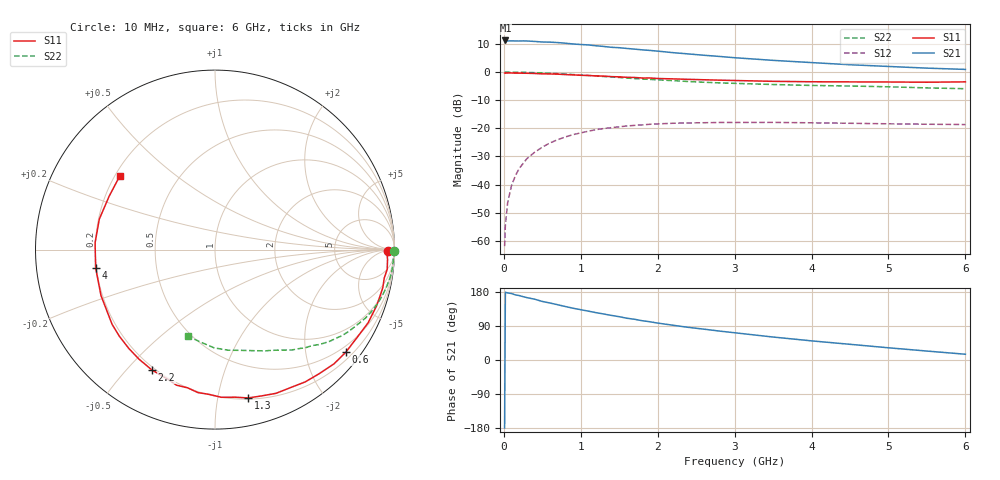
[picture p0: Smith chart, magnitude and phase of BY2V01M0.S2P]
! SIEMENS Small Signal Semiconductors
! BFY420
! Si NPN RF SIEGET Grounded Emitter Transistor in MICRO-X
! VCE = 2 V  IC = 1 mA
! Common Emitter S-Parameters:  October  1996
# GHz  S  MA  R  50
!  f  S11  S21  S12  S22
! GHz  MAG  ANG  MAG  ANG  MAG  ANG  MAG  ANG
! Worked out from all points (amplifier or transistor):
!   36 points, 10 MHz to 6 GHz, reference 50 ohm
!   highest |S21| = 11.3 dB at 20 MHz (marker M1)
!   |S21| within 3 dB of that: start of sweep to 1.666 GHz
!   unconditionally stable (mu >= 1): 4.55 GHz to end of sweep
!   at 250 MHz: K = 0.05, MSG = 21.8 dB, |S12| = -32.5 dB
!   at 1.4 GHz: K = 0.21, MSG = 14.3 dB, |S12| = -19.8 dB
!   at 6 GHz: K = 1.33, MAG = 6.4 dB, |S12| = -18.7 dB
!   S11 on the Smith chart (normalised r, x): 10 MHz: 48, -13; 600 MHz: 0.36, -2.86; 1.3 GHz: 0.21, -1.23; 2.2 GHz: 0.19, -0.59; 4 GHz: 0.20, -0.07; 6 GHz: 0.22, +0.32
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0.01  0.9622 -0.6  3.652 -179.3  0.0008 102.8  0.9999 -0.4
0.02  0.9583 -1.4  3.654 178.7  0.0019 88.0  0.9964 -0.6
0.05  0.9628 -3.2  3.583 177.0  0.0048 86.9  0.9983 -1.6
0.1  0.9657 -6.5  3.595 175.4  0.0096 85.8  0.9941 -3.2
0.15  0.9561 -9.6  3.579 171.8  0.0143 83.1  0.9947 -4.9
0.2  0.9588 -12.8  3.574 170.0  0.0193 81.8  0.9936 -6.3
0.3  0.9531 -19.2  3.574 164.6  0.0289 78.7  0.9866 -9.5
0.4  0.9457 -25.5  3.511 160.5  0.0374 74.2  0.977 -12.6
0.5  0.9306 -31.9  3.432 154.5  0.0462 70.5  0.9663 -15.6
0.6  0.9262 -38.1  3.409 150.4  0.055 67.0  0.9535 -18.6
0.8  0.9027 -50.0  3.265 141.1  0.0702 59.3  0.9222 -24.3
1.1  0.8699 -67.0  3.041 128.9  0.0889 49.8  0.8708 -31.8
1.3  0.8469 -77.4  2.858 121.3  0.0991 43.8  0.8347 -36.3
1.6  0.807 -92.4  2.633 110.2  0.1101 35.9  0.7835 -42.5
1.8  0.7851 -101.2  2.484 103.6  0.1151 31.2  0.7531 -45.8
2.2  0.7571 -117.7  2.216 91.7  0.1229 23.1  0.7048 -52.5
2.8  0.7189 -137.9  1.9 76.4  0.1269 14.1  0.6425 -60.9
3.5  0.6849 -158.0  1.617 60.6  0.1273 6.4  0.6011 -69.5
4  0.6729 -171.2  1.476 50.5  0.1253 2.7  0.5787 -75.9
4.5  0.6692 176.7  1.351 41.4  0.1228 -0.6  0.5654 -82.5
5.5  0.6605 153.2  1.176 23.6  0.1181 -3.0  0.5233 -98.1
6  0.67 142.5  1.116 15.2  0.1166 -2.6  0.5061 -107.0
